ORGANIZATION_BLOCK OB 1
BEGIN
	CALL		FC 1
	CALL		FC 2
END_ORGANIZATION_BLOCK



FUNCTION FC 1: VOID
BEGIN
	U		E 0.0
	=		A 0.0
END_FUNCTION



FUNCTION FC 2: VOID
TITLE = Shift register
BEGIN
	UN		T 10
	=		M 0.0
	L		S5T#200MS
	SV		T 10

	L		MD 4
	L		1
	==D
	S		M 0.1
	RRD		1
	==D
	R		M 0.1

	L		MD 4
	UD		L#-1
	L		1
	SPZ		_001
	TAK
	U		M 0.0
	SPBN		_001
	U		M 0.1
	SPBN		_000
	RLD		2
_000:	RRD		1
_001:	T		MD 4

	L		MD 4
	T		AD 4
	TAD
	T		AD 8
END_FUNCTION
